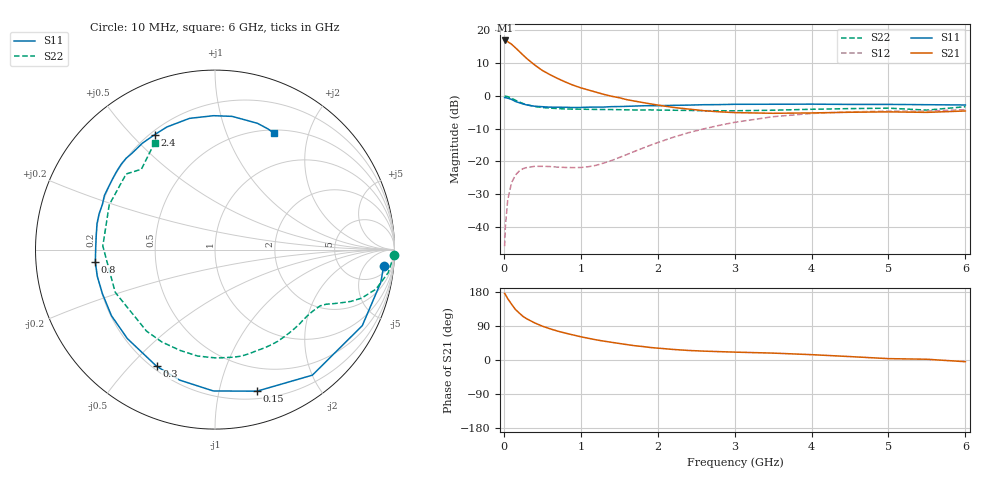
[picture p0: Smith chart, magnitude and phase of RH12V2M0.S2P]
! SIEMENS Small Signal Semiconductors
! BFR106
! Si NPN RF Bipolar Junction Transistor in SOT23
! VCE = 12 V  IC = 2 mA
! Common Emitter S-Parameters:  August  1996
# GHz  S  MA  R  50
!  f  S11  S21  S12  S22
! GHz  MAG  ANG  MAG  ANG  MAG  ANG  MAG  ANG
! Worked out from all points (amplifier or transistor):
!   36 points, 10 MHz to 6 GHz, reference 50 ohm
!   highest |S21| = 16.9 dB at 20 MHz (marker M1)
!   |S21| within 3 dB of that: start of sweep to 185.4 MHz
!   unconditionally stable (mu >= 1): 786 MHz to 1.799 GHz; 4.192 GHz to end of sweep
!   at 250 MHz: K = 0.32, MSG = 17.3 dB, |S12| = -22.2 dB
!   at 1.4 GHz: K = 1.24, MAG = 6.9 dB, |S12| = -19.7 dB
!   at 6 GHz: K = 1.02, MAG = -1.1 dB, |S12| = -4.2 dB
!   S11 on the Smith chart (normalised r, x): 10 MHz: 9, -15; 150 MHz: 0.27, -1.30; 300 MHz: 0.22, -0.60; 800 MHz: 0.20, -0.05; 2.4 GHz: 0.22, +0.58; 6 GHz: 0.54, +1.49
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0.01  0.9443 -5.4  7.01 175.7  0.0051 89.2  0.9988 -1.6
0.02  0.9417 -11.2  7.013 173.0  0.0101 86.9  0.9912 -3.1
0.05  0.9235 -27.3  6.719 162.0  0.0257 74.7  0.9736 -7.6
0.1  0.8853 -52.2  6.153 147.4  0.0473 63.0  0.9235 -13.8
0.15  0.8227 -73.5  5.434 133.5  0.0618 52.0  0.8604 -18.3
0.2  0.7876 -90.7  4.784 123.9  0.0714 44.9  0.8095 -20.9
0.25  0.7532 -105.2  4.193 114.9  0.0777 38.9  0.7641 -22.8
0.3  0.7268 -116.6  3.701 108.5  0.0808 35.7  0.7326 -24.2
0.4  0.6959 -134.6  2.967 98.0  0.0842 30.5  0.6896 -26.2
0.5  0.6844 -147.5  2.448 89.3  0.0843 28.5  0.6649 -28.1
0.6  0.6736 -158.5  2.108 82.4  0.0837 28.6  0.6511 -30.5
0.8  0.6704 -174.1  1.629 71.0  0.081 33.3  0.6329 -35.8
1.1  0.6731 167.6  1.229 57.2  0.0832 48.6  0.624 -45.2
1.6  0.6931 145.6  0.876 40.6  0.1276 71.1  0.6131 -63.3
2.2  0.7177 124.3  0.668 27.9  0.2334 73.1  0.6043 -89.1
2.4  0.7235 117.6  0.63 25.2  0.2744 70.3  0.6009 -99.3
3  0.7448 101.0  0.556 20.8  0.3953 57.7  0.5931 -130.0
3.5  0.7461 90.6  0.543 18.2  0.4818 45.4  0.6048 -156.8
4.5  0.7417 76.6  0.563 9.0  0.5707 22.1  0.6399 157.1
5  0.7422 71.4  0.571 3.6  0.586 13.0  0.6502 139.6
5.5  0.7343 66.2  0.561 2.0  0.5856 8.4  0.6072 132.5
6  0.7267 63.2  0.589 -4.5  0.6171 0.1  0.6838 119.5
